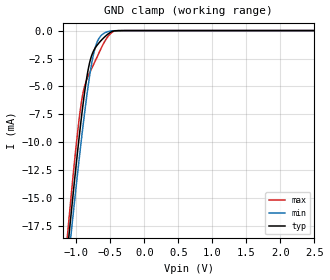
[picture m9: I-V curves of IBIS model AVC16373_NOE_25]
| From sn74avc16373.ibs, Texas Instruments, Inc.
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[Model]   AVC16373_NOE_25
Model_type  Input
Vinl=0.7
Vinh=1.7
| variable   typ   min   max
C_comp   1.85pF   1.32pF   2.42pF
[Temperature Range]   40   100   -40
| Ambient temperature   25   85   -40
[Voltage range]   2.5   2.3   2.7
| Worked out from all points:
|   GND clamp passes 1 mA (typ) near -0.65 V on its own axis
[GND Clamp]
| AVC16373_NOE_25
|   Voltage   I(typ)   I(min)   I(max)
-2.5V     -112.2mA   -109.4mA   -117.8mA
-1.135V   -19.94mA   -21.57mA   -18.57mA
-1.1V     -17.78mA   -19.5mA    -16.27mA
-1.07V    -15.95mA   -17.74mA   -14.34mA
-935mV    -8.251mA   -10.21mA   -6.785mA
-885mV    -5.791mA   -7.647mA   -5.114mA
-825mV    -3.443mA   -4.871mA   -4.055mA
-715mV    -1.48mA    -1.36mA    -2.619mA
-595mV    -630.8uA   -252uA     -1.097mA
-485mV    -114.4uA   -29.54uA   -203.1uA
-380mV    -5.562uA   -4.599uA   -5.667uA
2.5V      206.6pA    685.3pA    11.37pA
